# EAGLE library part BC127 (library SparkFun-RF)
Blue Creations BC127 BLE module The BC127 is a highly flexible, low power, small form factor Bluetooth Version 4.0 Certified Audio module. It comes preloaded with BlueCreation Melody software, and is ideal for developers who want to quickly and cost effectively integrate Bluetooth functionality into their products. SparkFun Products: Bluetooth SMD Module - BC127 (WRL-12819) Bluetooth Audio Breakout - BC127 (WRL-11927) Purpletooth Jamboree - BC127 Development Board (WRL-11924)
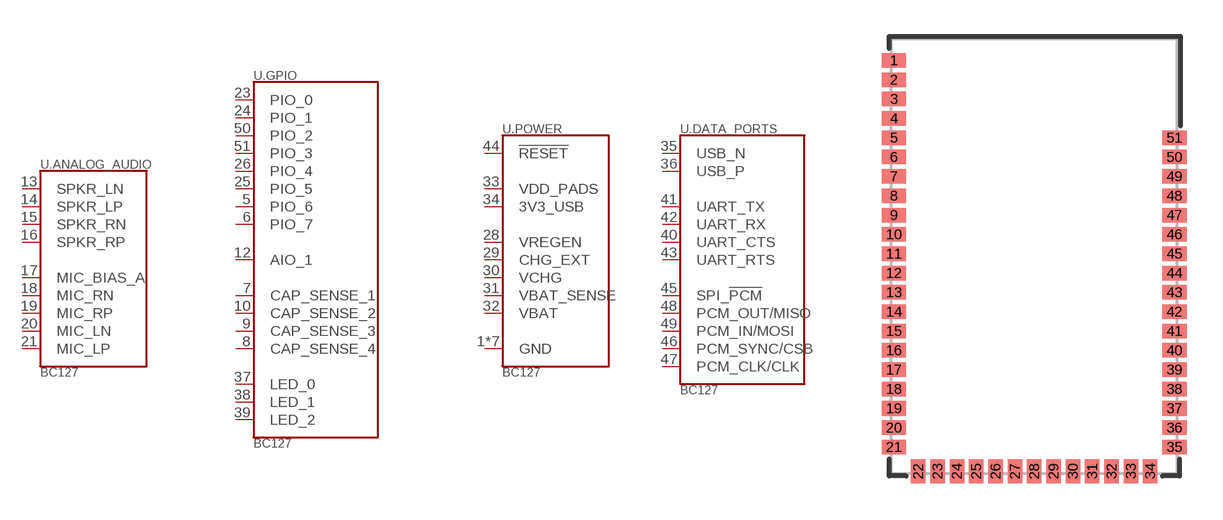
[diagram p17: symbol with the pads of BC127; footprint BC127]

Designator prefix U; gates .ANALOG_AUDIO=BC127_ANALOG_AUDIO .GPIO=BC127_GPIO .POWER=BC127_POWER .DATA_PORTS=BC127_DATA_PORTS

## BC127" (PROD_ID: IC-11659)  [BC127]
1  .POWER:GND
2  .POWER:GND
3  .POWER:GND
4  .POWER:GND
5  .GPIO:PIO_6
6  .GPIO:PIO_7
7  .GPIO:CAP_SENSE_1
8  .GPIO:CAP_SENSE_4
9  .GPIO:CAP_SENSE_3
10  .GPIO:CAP_SENSE_2
11  .POWER:GND
12  .GPIO:AIO_1
13  .ANALOG_AUDIO:SPKR_LN
14  .ANALOG_AUDIO:SPKR_LP
15  .ANALOG_AUDIO:SPKR_RN
16  .ANALOG_AUDIO:SPKR_RP
17  .ANALOG_AUDIO:MIC_BIAS_A
18  .ANALOG_AUDIO:MIC_RN
19  .ANALOG_AUDIO:MIC_RP
20  .ANALOG_AUDIO:MIC_LN
21  .ANALOG_AUDIO:MIC_LP
22  .POWER:GND
23  .GPIO:PIO_0
24  .GPIO:PIO_1
25  .GPIO:PIO_5
26  .GPIO:PIO_4
27  .POWER:GND
28  .POWER:VREGEN
29  .POWER:CHG_EXT
30  .POWER:VCHG
31  .POWER:VBAT_SENSE
32  .POWER:VBAT
33  .POWER:VDD_PADS
34  .POWER:3V3_USB
35  .DATA_PORTS:USB_N
36  .DATA_PORTS:USB_P
37  .GPIO:LED_0
38  .GPIO:LED_1
39  .GPIO:LED_2
40  .DATA_PORTS:UART_CTS
41  .DATA_PORTS:UART_TX
42  .DATA_PORTS:UART_RX
43  .DATA_PORTS:UART_RTS
44  .POWER:!RESET
45  .DATA_PORTS:SPI_!PCM
46  .DATA_PORTS:PCM_SYNC/CSB
47  .DATA_PORTS:PCM_CLK/CLK
48  .DATA_PORTS:PCM_OUT/MISO
49  .DATA_PORTS:PCM_IN/MOSI
50  .GPIO:PIO_2
51  .GPIO:PIO_3

## Footprint BC127 (pad centres in mm)
BC127 Bluetooth 4.0 Audio Module 11.8x18mm module. Extra tCream on pads. Datasheet
smd 1 x 0.6: 1 -5.8,8.1; 2 -5.8,7.3; 3 -5.8,6.5; 4 -5.8,5.7; 5 -5.8,4.9; 6 -5.8,4.1; 7 -5.8,3.3; 8 -5.8,2.5; 9 -5.8,1.7; 10 -5.8,0.9; 11 -5.8,0.1; 12 -5.8,-0.7; 13 -5.8,-1.5; 14 -5.8,-2.3; 15 -5.8,-3.1; 16 -5.8,-3.9; 17 -5.8,-4.7; 18 -5.8,-5.5; 19 -5.8,-6.3; 20 -5.8,-7.1; 21 -5.8,-7.9; 35 5.8,-7.9; 36 5.8,-7.1; 37 5.8,-6.3; 38 5.8,-5.5; 39 5.8,-4.7; 40 5.8,-3.9; 41 5.8,-3.1; 42 5.8,-2.3; 43 5.8,-1.5; 44 5.8,-0.7; 45 5.8,0.1; 46 5.8,0.9; 47 5.8,1.7; 48 5.8,2.5; 49 5.8,3.3; 50 5.8,4.1; 51 5.8,4.9
smd 0.6 x 1: 22 -4.8,-8.9; 23 -4,-8.9; 24 -3.2,-8.9; 25 -2.4,-8.9; 26 -1.6,-8.9; 27 -0.8,-8.9; 28 0,-8.9; 29 0.8,-8.9; 30 1.6,-8.9; 31 2.4,-8.9; 32 3.2,-8.9; 33 4,-8.9; 34 4.8,-8.9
